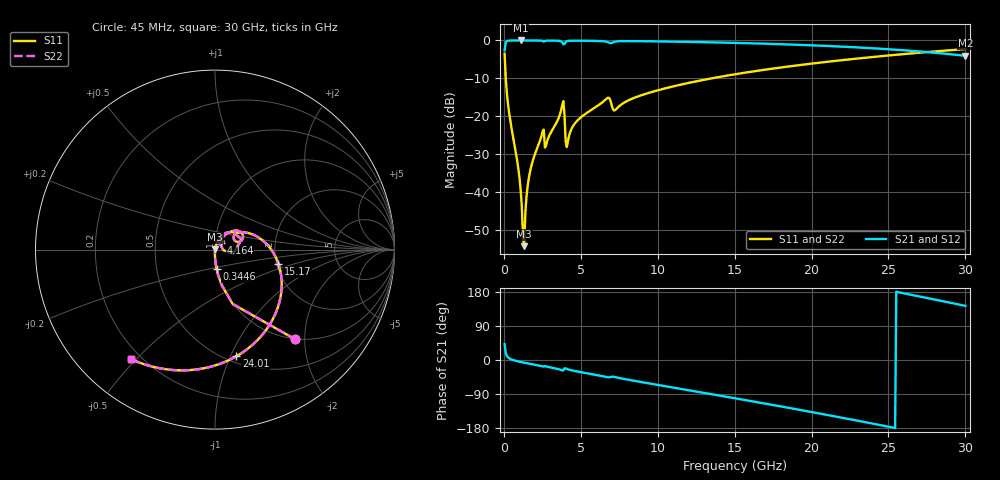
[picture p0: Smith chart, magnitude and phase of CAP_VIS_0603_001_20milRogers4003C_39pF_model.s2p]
! S-parameter model data by Modelithics Inc.  support@modelithics.com  813-866-6335  Tampa FL USA
! S-Parameter data specifications:
! Substrate: 20-mil Rogers 4003C, substrate thickness, H=0.508mm, Dielectric constant, Er=3.75
! PCB Mounting Pad Footprint: Pad width, PadW=0.90mm , Pad length, PadL=1.00mm , Pad gap, PadG (edge-to-edge)=1.00mm , Reference planes=3.0mm apart
! Created Wed Nov 18 13:28:29 2015
# hz S ma R 50
! 2 Port Network Data from SP1.SP block
! freq  magS11  angS11  magS21  angS21  magS12  angS12  magS22  angS22
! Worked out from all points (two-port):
!   401 points, 45 MHz to 30 GHz, reference 50 ohm
!   highest |S21| = -0.01 dB at 1.093 GHz (marker M1); lowest = -4.0 dB at 30 GHz (marker M2)
!   |S21| within 3 dB of the highest: start of sweep to 27.32 GHz
!   lowest |S11| = -54.2 dB at 1.318 GHz (marker M3), VSWR 1.00, Z = 50.1 + j0.148 ohm
!   |S11| at or under -10 dB: 120.9 MHz to 13.49 GHz (13.37 GHz wide, 196 % of centre)
!   |S22| runs from -54.2 to -2.3 dB; largest |S21 - S12| = 0
!   S11 on the Smith chart (normalised r, x): 45 MHz: 0.99, -1.80; 344.6 MHz: 0.99, -0.22; 4.164 GHz: 1.06, +0.08; 15.17 GHz: 2.05, -0.37; 24.01 GHz: 0.56, -1.05; 30 GHz: 0.16, -0.48
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4.5e7  0.6693 -48.2  0.7428 41.8  0.7428 41.8  0.6693 -48.2
3.4455e8  0.1088 -85.3  0.9935 4.4  0.9935 4.4  0.1088 -85.3
8.687625e8  0.0256 -91.2  0.9987 -3.1  0.9987 -3.1  0.0256 -91.2
1.093425e9  0.01046 -89.8  0.9989 -5.2  0.9989 -5.2  0.01046 -89.8
1.168312e9  0.006227 -86.5  0.9989 -5.9  0.9989 -5.9  0.006227 -86.5
1.318088e9  0.001948 49.3  0.9988 -7.1  0.9988 -7.1  0.001948 49.3
1.392975e9  0.005332 70.3  0.9988 -7.7  0.9988 -7.7  0.005332 70.3
1.692525e9  0.01842 76.0  0.9984 -10.0  0.9984 -10.0  0.01842 76.0
2.4414e9  0.05491 68.7  0.9933 -16.1  0.9933 -16.1  0.05491 68.7
2.815838e9  0.04735 66.3  0.9936 -17.6  0.9936 -17.6  0.04735 66.3
3.789375e9  0.1403 44.4  0.9478 -27.8  0.9478 -27.8  0.1403 44.4
4.163812e9  0.04757 48.5  0.9848 -24.7  0.9848 -24.7  0.04757 48.5
5.062462e9  0.09914 55.5  0.9912 -32.5  0.9912 -32.5  0.09914 55.5
6.709988e9  0.1732 34.7  0.9548 -45.4  0.9548 -45.4  0.1732 34.7
7.2342e9  0.1209 31.2  0.9637 -45.1  0.9637 -45.1  0.1209 31.2
1.007992e10  0.2224 22.8  0.9703 -66.3  0.9703 -66.3  0.2224 22.8
1.50225e10  0.3581 -11.6  0.9283 -101.0  0.9283 -101.0  0.3581 -11.6
1.517228e10  0.3622 -12.6  0.9267 -102.0  0.9267 -102.0  0.3622 -12.6
2.003996e10  0.496 -48.1  0.8617 -137.6  0.8617 -137.6  0.496 -48.1
2.4009e10  0.6058 -78.6  0.7876 -168.1  0.7876 -168.1  0.6058 -78.6
2.505742e10  0.6349 -86.9  0.7641 -176.5  0.7641 -176.5  0.6349 -86.9
3e10  0.769 -127.5  0.6282 142.9  0.6282 142.9  0.769 -127.5
